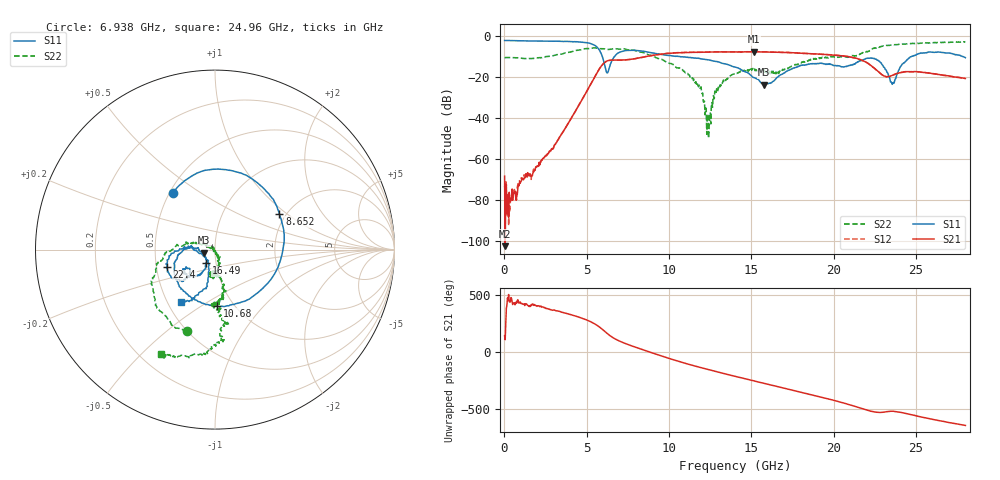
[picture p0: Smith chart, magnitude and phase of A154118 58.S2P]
!  2-Port S-parameters saved by WinCal
! VAR MeasName=S-Parameters (CALIBRATED_DATA) read from VNA (N5230A)
! VAR MeasDate=2015-9-10 14:39:35
! VAR NAME=A154118 58
! VAR FILENAME=A154118 58.S2P
! VAR DATE=2015-9-10 14:39:35
! VAR PHYS_PORTS=1,2
# Hz S DB R 50
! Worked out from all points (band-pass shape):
!   801 points, 10 MHz to 28 GHz, reference 50 ohm
!   highest |S21| = -7.65 dB at 15.16 GHz (marker M1); lowest = -102.5 dB at 44.99 MHz (marker M2)
!   |S21| within 3 dB of the highest: 8.162 GHz to 21.29 GHz (13.12 GHz wide, 89.1 % of centre)
!   lowest |S11| = -23.8 dB at 15.75 GHz (marker M3), VSWR 1.14, Z = 44.1 - j1.55 ohm
!   |S11| at or under -10 dB: 5.946 GHz to 6.682 GHz (736 MHz wide, 11.7 % of centre); 10.66 GHz to 24.72 GHz (14.06 GHz wide, 79.5 % of centre); 27.86259 GHz to end of sweep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
!   |S22| runs from -49.8 to -2.7 dB; largest |S21 - S12| = 0.008
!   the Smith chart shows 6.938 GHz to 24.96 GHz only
!   S11 on the Smith chart (normalised r, x): 6.938 GHz: 0.52, +0.39; 8.652 GHz: 1.85, +0.88; 10.68 GHz: 0.84, -0.58; 16.49 GHz: 0.89, -0.14; 22.4 GHz: 0.57, -0.12; 24.96 GHz: 0.59, -0.39
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1e7  -2.15 179.7  -68.39 140.2  -73.30 -80.0  -10.60 179.8
4.49875e7  -2.14 179.3  -102.54 106.7  -77.41 37.4  -10.53 178.3
6.39775e8  -2.26 171.0  -75.72 53.5  -76.91 48.8  -10.57 151.6
4.698325e9  -3.01 98.3  -31.31 -64.0  -31.29 -64.5  -6.55 -29.5
5.677975e9  -5.87 37.2  -17.15 -132.3  -17.13 -132.4  -5.95 -71.0
6.132812e9  -15.63 -50.1  -12.61 174.3  -12.62 174.3  -6.38 -85.8
6.937525e9  -8.11 126.4  -11.72 98.1  -11.74 97.9  -6.35 -108.9
8.651912e9  -7.73 29.0  -9.91 7.0  -9.89 7.2  -8.80 -158.1
9.351662e9  -8.72 -13.4  -9.03 -27.2  -8.99 -27.0  -10.94 -174.5
1.068119e10  -10.06 -88.1  -8.14 -87.7  -8.05 -88.1  -15.81 165.5
1.190575e10  -11.03 -136.5  -7.92 -137.0  -7.85 -137.6  -25.36 146.4
1.239558e10  -11.66 -149.8  -7.81 -155.8  -7.74 -156.4  -49.81 -79.4
1.281542e10  -12.38 -159.9  -7.74 -171.3  -7.70 -171.9  -27.06 -55.0
1.4005e10  -15.12 179.8  -7.75 145.7  -7.76 145.0  -18.34 -85.6
1.515959e10  -20.28 174.3  -7.65 105.6  -7.66 104.9  -16.09 -97.4
1.575438e10  -23.75 -164.4  -7.77 84.0  -7.75 83.6  -17.51 -100.6
1.648911e10  -20.81 -123.4  -7.91 58.7  -7.85 58.1  -17.60 -90.7
1.869332e10  -13.43 -135.6  -8.64 -17.9  -8.68 -18.5  -11.00 -80.8
2.2402e10  -10.91 -160.0  -15.26 -164.8  -15.29 -166.0  -5.94 -85.8
2.334666e10  -19.76 -176.9  -19.78 -162.7  -19.82 -163.8  -4.56 -99.6
2.495609e10  -9.24 -123.1  -17.33 160.9  -17.36 160.6  -3.67 -117.2
2.8e10  -10.56 171.8  -20.70 74.4  -20.71 74.1  -2.74 -140.6
